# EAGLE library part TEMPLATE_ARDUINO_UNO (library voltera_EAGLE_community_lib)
Use SHIELD for integrating into circuits. Use RAW for created the template boards.
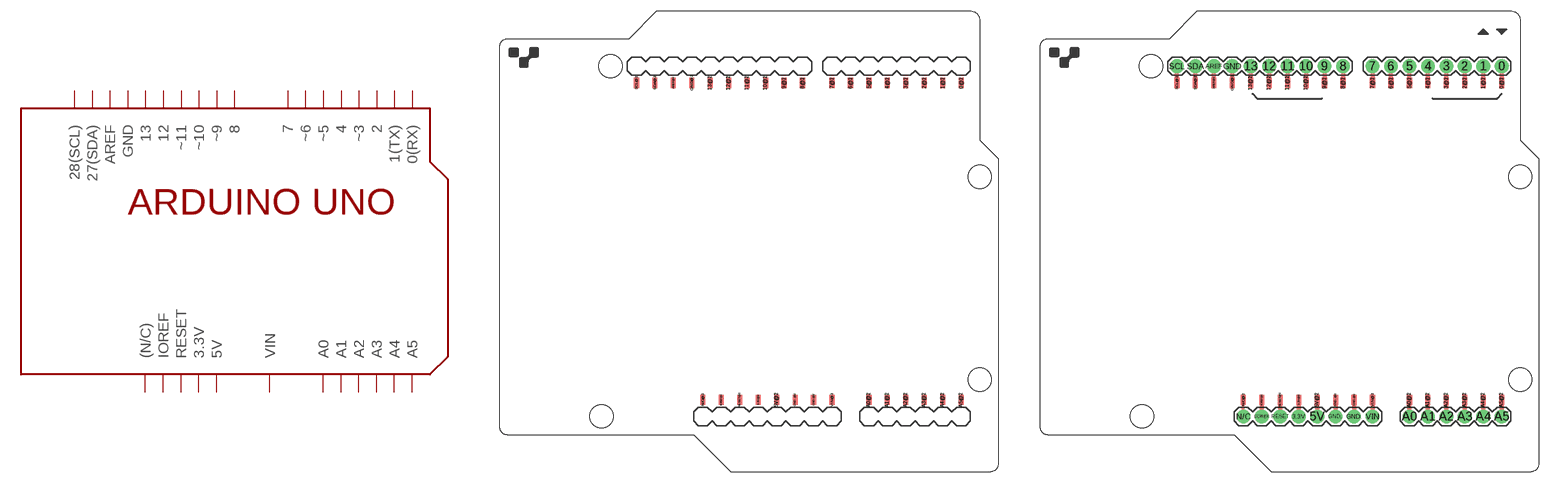
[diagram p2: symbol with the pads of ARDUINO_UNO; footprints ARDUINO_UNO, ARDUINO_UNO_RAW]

Designator prefix -

## TEMPLATE_ARDUINO_UNO_SHIELD  [ARDUINO_UNO]
0@1  0(RX)
0@2  0(RX)
1@1  1(TX)
1@2  1(TX)
2@1  2
2@2  2
3.3V@1  3.3V
3.3V@2  3.3V
3@1  ~3
3@2  ~3
4@1  4
4@2  4
5@1  ~5
5@2  ~5
5V@1  5V
5V@2  5V
6@1  ~6
6@2  ~6
7@1  7
7@2  7
8@1  8
8@2  8
9@1  ~9
9@2  ~9
10@1  ~10
10@2  ~10
11@1  ~11
11@2  ~11
12@1  12
12@2  12
13@1  13
13@2  13
A0@1  A0
A0@2  A0
A1@1  A1
A1@2  A1
A2@1  A2
A2@2  A2
A3@1  A3
A3@2  A3
A4@1  A4
A4@2  A4
A5@1  A5
A5@2  A5
AREF@1  AREF
AREF@2  AREF
GND..@1  GND
GND..@2  GND
GND.@1  GND
GND.@2  GND
GND@1  GND
GND@2  GND
I/OREF@1  IOREF
I/OREF@2  IOREF
N/C@1  (N/C)
N/C@2  (N/C)
RESET@1  RESET
RESET@2  RESET
SCL@1  28(SCL)
SCL@2  28(SCL)
SDA@1  27(SDA)
SDA@2  27(SDA)
VIN@1  VIN
VIN@2  VIN

## TEMPLATE_ARDUINO_UNO_RAW  [ARDUINO_UNO_RAW]
0  0(RX)
0@1  0(RX)
0@2  0(RX)
1  1(TX)
1@1  1(TX)
1@2  1(TX)
2  2
2@1  2
2@2  2
3  ~3
3.3V  3.3V
3.3V@1  3.3V
3.3V@2  3.3V
3@1  ~3
3@2  ~3
4  4
4@1  4
4@2  4
5  ~5
5@1  ~5
5@2  ~5
5V  5V
5V@1  5V
5V@2  5V
6  ~6
6@1  ~6
6@2  ~6
7  7
7@1  7
7@2  7
8  8
8@1  8
8@2  8
9  ~9
9@1  ~9
9@2  ~9
10  ~10
10@1  ~10
10@2  ~10
11  ~11
11@1  ~11
11@2  ~11
12  12
12@1  12
12@2  12
13  13
13@1  13
13@2  13
A0  A0
A0@1  A0
A0@2  A0
A1  A1
A1@1  A1
A1@2  A1
A2  A2
A2@1  A2
A2@2  A2
A3  A3
A3@1  A3
A3@2  A3
A4  A4
A4@1  A4
A4@2  A4
A5  A5
A5@1  A5
A5@2  A5
AREF  AREF
AREF@1  AREF
AREF@2  AREF
GND  GND
GND.  GND
GND..  GND
GND..@1  GND
GND..@2  GND
GND.@1  GND
GND.@2  GND
GND@1  GND
GND@2  GND
I/OREF  IOREF
I/OREF@1  IOREF
I/OREF@2  IOREF
N/C  (N/C)
N/C@1  (N/C)
N/C@2  (N/C)
RESET  RESET
RESET@1  RESET
RESET@2  RESET
SCL  28(SCL)
SCL@1  28(SCL)
SCL@2  28(SCL)
SDA  27(SDA)
SDA@1  27(SDA)
SDA@2  27(SDA)
VIN  VIN
VIN@1  VIN
VIN@2  VIN

## Footprint ARDUINO_UNO (pad centres in mm)
smd 0.711 x 1.422 bottom: 0@1 30.48,23.114; 1@1 27.94,23.114; 2@1 25.4,23.114; 3.3V@1 2.54,-20.574; 3@1 22.86,23.114; 4@1 20.32,23.114; 5@1 17.78,23.114; 5V@1 5.08,-20.574; 6@1 15.24,23.114; 7@1 12.7,23.114; 8@1 8.636,23.114; 9@1 6.096,23.114; 10@1 3.556,23.114; 11@1 1.016,23.114; 12@1 -1.524,23.114; 13@1 -4.064,23.114; A0@1 17.78,-20.574; A1@1 20.32,-20.574; A2@1 22.86,-20.574; A3@1 25.4,-20.574; A4@1 27.94,-20.574; A5@1 30.48,-20.574; AREF@1 -9.144,23.114; GND..@1 7.62,-20.574; GND.@1 10.16,-20.574; GND@1 -6.604,23.114; I/OREF@1 -2.54,-20.574; N/C@1 -5.08,-20.574; RESET@1 0,-20.574; SCL@1 -14.224,23.114; SDA@1 -11.684,23.114; VIN@1 12.7,-20.574
smd 0.711 x 1.422: 0@2 30.48,23.114; 1@2 27.94,23.114; 2@2 25.4,23.114; 3.3V@2 2.54,-20.574; 3@2 22.86,23.114; 4@2 20.32,23.114; 5@2 17.78,23.114; 5V@2 5.08,-20.574; 6@2 15.24,23.114; 7@2 12.7,23.114; 8@2 8.636,23.114; 9@2 6.096,23.114; 10@2 3.556,23.114; 11@2 1.016,23.114; 12@2 -1.524,23.114; 13@2 -4.064,23.114; A0@2 17.78,-20.574; A1@2 20.32,-20.574; A2@2 22.86,-20.574; A3@2 25.4,-20.574; A4@2 27.94,-20.574; A5@2 30.48,-20.574; AREF@2 -9.144,23.114; GND..@2 7.62,-20.574; GND.@2 10.16,-20.574; GND@2 -6.604,23.114; I/OREF@2 -2.54,-20.574; N/C@2 -5.08,-20.574; RESET@2 0,-20.574; SCL@2 -14.224,23.114; SDA@2 -11.684,23.114; VIN@2 12.7,-20.574
hole 3.2 at 33.02,-17.78
hole 3.2 at 33.02,10.16
hole 3.2 at -17.78,25.4
hole 3.2 at -19.05,-22.86

## Footprint ARDUINO_UNO_RAW (pad centres in mm)
drill 1.016 pad 1.88: 0 29.21,25.4; 1 26.67,25.4; 2 24.13,25.4; 3 21.59,25.4; 3.3V 1.27,-22.86; 4 19.05,25.4; 5 16.51,25.4; 5V 3.81,-22.86; 6 13.97,25.4; 7 11.43,25.4; 8 7.366,25.4; 9 4.826,25.4; 10 2.286,25.4; 11 -0.254,25.4; 12 -2.794,25.4; 13 -5.334,25.4; A0 16.51,-22.86; A1 19.05,-22.86; A2 21.59,-22.86; A3 24.13,-22.86; A4 26.67,-22.86; A5 29.21,-22.86; AREF -10.414,25.4; GND -7.874,25.4; GND. 8.89,-22.86; GND.. 6.35,-22.86; I/OREF -3.81,-22.86; N/C -6.35,-22.86; RESET -1.27,-22.86; SCL -15.494,25.4; SDA -12.954,25.4; VIN 11.43,-22.86
smd 0.711 x 1.422 bottom: 0@1 29.21,23.114; 1@1 26.67,23.114; 2@1 24.13,23.114; 3.3V@1 1.27,-20.574; 3@1 21.59,23.114; 4@1 19.05,23.114; 5@1 16.51,23.114; 5V@1 3.81,-20.574; 6@1 13.97,23.114; 7@1 11.43,23.114; 8@1 7.366,23.114; 9@1 4.826,23.114; 10@1 2.286,23.114; 11@1 -0.254,23.114; 12@1 -2.794,23.114; 13@1 -5.334,23.114; A0@1 16.51,-20.574; A1@1 19.05,-20.574; A2@1 21.59,-20.574; A3@1 24.13,-20.574; A4@1 26.67,-20.574; A5@1 29.21,-20.574; AREF@1 -10.414,23.114; GND..@1 6.35,-20.574; GND.@1 8.89,-20.574; GND@1 -7.874,23.114; I/OREF@1 -3.81,-20.574; N/C@1 -6.35,-20.574; RESET@1 -1.27,-20.574; SCL@1 -15.494,23.114; SDA@1 -12.954,23.114; VIN@1 11.43,-20.574
smd 0.711 x 1.422: 0@2 29.21,23.114; 1@2 26.67,23.114; 2@2 24.13,23.114; 3.3V@2 1.27,-20.574; 3@2 21.59,23.114; 4@2 19.05,23.114; 5@2 16.51,23.114; 5V@2 3.81,-20.574; 6@2 13.97,23.114; 7@2 11.43,23.114; 8@2 7.366,23.114; 9@2 4.826,23.114; 10@2 2.286,23.114; 11@2 -0.254,23.114; 12@2 -2.794,23.114; 13@2 -5.334,23.114; A0@2 16.51,-20.574; A1@2 19.05,-20.574; A2@2 21.59,-20.574; A3@2 24.13,-20.574; A4@2 26.67,-20.574; A5@2 29.21,-20.574; AREF@2 -10.414,23.114; GND..@2 6.35,-20.574; GND.@2 8.89,-20.574; GND@2 -7.874,23.114; I/OREF@2 -3.81,-20.574; N/C@2 -6.35,-20.574; RESET@2 -1.27,-20.574; SCL@2 -15.494,23.114; SDA@2 -12.954,23.114; VIN@2 11.43,-20.574
hole 3.2 at 31.75,-17.78
hole 3.2 at 31.75,10.16
hole 3.2 at -19.05,25.4
hole 3.2 at -20.32,-22.86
